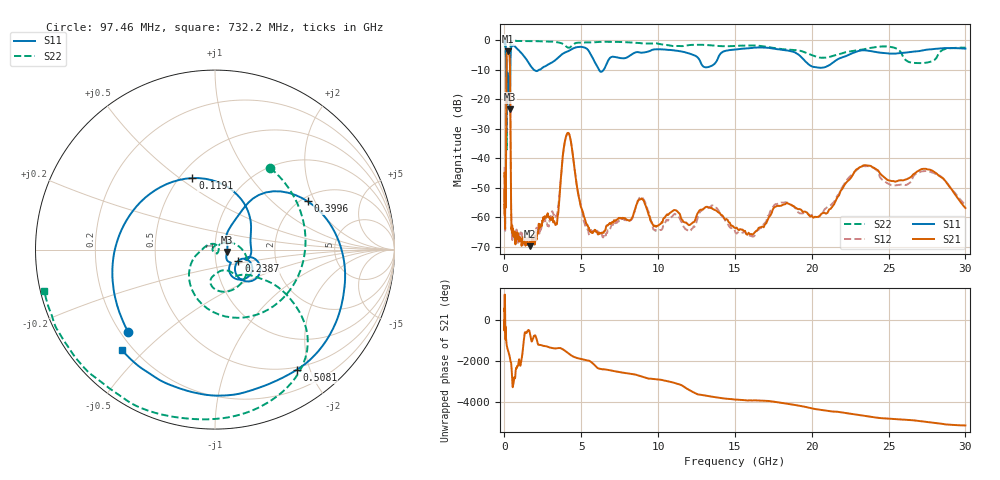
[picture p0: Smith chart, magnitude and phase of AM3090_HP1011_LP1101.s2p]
! Date/Time: Thu, Feb 28, 2019 2:06 PM
! Network Analyzer: Agilent Technologies E8364B Rev: A.07.50.67
! Sweep from 0.010 to 30.000 GHz, 1601 Points, Sweep Type: LOG
! Power Supply: 5.023 V, 0.002 A
# Hz S DB R 50
!freq MagS11 AngS11 MagS21 AngS21 MagS12 AngS12 MagS22 AngS22
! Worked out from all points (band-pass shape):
!   1601 points, 10 MHz to 30 GHz, reference 50 ohm
!   highest |S21| = -3.77 dB at 238.7 MHz (marker M1); lowest = -69.8 dB at 1.647 GHz (marker M2)
!   |S21| within 3 dB of the highest: 132.8 MHz to 347.9 MHz (215.1 MHz wide, 89.5 % of centre)
!   lowest |S11| = -23.4 dB at 340.5 MHz (marker M3), VSWR 1.15, Z = 57.1 - j1.47 ohm
!   |S11| at or under -10 dB: 124.6 MHz to 381.7 MHz (257.1 MHz wide, 102 % of centre); 1.899 GHz to 2.277 GHz (377.8 MHz wide, 18.1 % of centre); 6.145 GHz to 6.463 GHz (318 MHz wide, 5.04 % of centre)
!   |S22| runs from -37.1 to -0.1 dB; largest |S21 - S12| = 0.012
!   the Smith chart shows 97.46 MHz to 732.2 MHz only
!   S11 on the Smith chart (normalised r, x): 97.46 MHz: 0.23, -0.38; 119.1 MHz: 0.58, +0.56; 238.7 MHz: 1.29, -0.16; 399.6 MHz: 2.16, +1.76; 508.1 MHz: 0.46, -1.80; 732.2 MHz: 0.16, -0.43
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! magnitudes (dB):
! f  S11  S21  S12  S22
! 10 MHz  -0.3  -46.2  -42.9  -0.7
! 38.04 MHz  -0.4  -59.9  -58.1  -1.6
! 97.46 MHz  -3.5  -52.9  -51.2  -5.2
! 119.1 MHz  -7.6  -17.0  -17.0  -8.5
! 144.7 MHz  -13.9  -5.0  -5.0  -35.2
! 181.3 MHz  -12.0  -3.9  -3.9  -13.9
! 238.7 MHz  -16.8  -3.8  -3.7  -15.8
! 340.5 MHz  -23.4  -6.0  -6.0  -12.6
! 399.6 MHz  -4.7  -34.7  -34.7  -1.2
! 446.1 MHz  -2.4  -60.8  -61.3  -0.4
! 508.1 MHz  -1.8  -64.2  -67.2  -0.2
! 550.5 MHz  -1.8  -64.8  -66.8  -0.2
! 732.2 MHz  -2.3  -67.5  -66.9  -0.2
! 1.647 GHz  -8.3  -69.8  -68.3  -0.3
! 2.084 GHz  -10.5  -67.6  -63.5  -0.4
! 3.385 GHz  -6.4  -62.1  -59.6  -0.7
! 4.115 GHz  -3.8  -31.4  -31.5  -2.5
! 5.365 GHz  -2.9  -62.5  -63.8  -0.8
! 7.926 GHz  -6.0  -60.6  -60.9  -0.7
! 16.05 GHz  -2.7  -65.6  -66.2  -1.8
! 23.59 GHz  -3.5  -42.5  -42.6  -2.9
! 30 GHz  -2.9  -56.8  -55.9  -2.5
